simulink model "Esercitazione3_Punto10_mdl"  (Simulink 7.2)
settings: Solver=ode45  StartTime=0.0  StopTime=10.0  RelTol=1e-3
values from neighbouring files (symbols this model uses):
  A = [-6.1   15.4    1.6    [Esercitazione07.m]
  B = [1; 0; 0]    [Esercitazione07.m]
  C = [0 10 10]    [Esercitazione07.m]
  Kyu = -inv(C*inv(A-B*K)*B)    [Esercitazione07.m]
  L = - acker(A',C',[-4 -4 -4])'    [Esercitazione07.m]
  s1 = 5    [Esercitazione07.m]
  s2 = 20    [Esercitazione07.m]
  t1 = 0    [Esercitazione07.m]
  t2 = 10    [Esercitazione07.m]
  X0 = [7 -1 2]'    [Esercitazione07.m]
undefined symbols (not defined in the file or in its folder): K, sd, td

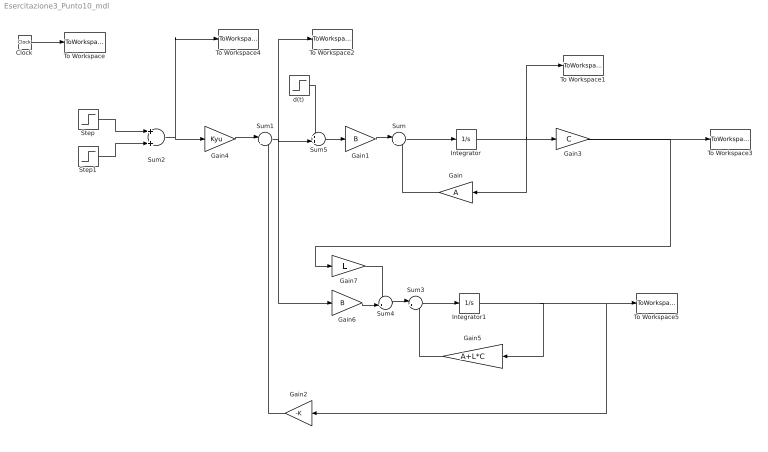
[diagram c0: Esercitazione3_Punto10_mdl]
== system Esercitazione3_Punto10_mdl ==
  Clock : Clock
  Gain : Gain  Orientation=left  Gain=A  Multiplication=Matrix(K*u)  ParameterDataType=sfix(16)  ParameterScaling=2^0  OutDataType=sfix(16)  OutScaling=2^0
  Gain1 : Gain  Gain=B  Multiplication=Matrix(K*u)  ParameterDataType=sfix(16)  ParameterScaling=2^0  OutDataType=sfix(16)  OutScaling=2^0
  Gain2 : Gain  Orientation=left  Gain=-K  Multiplication=Matrix(K*u)  ParameterDataType=sfix(16)  ParameterScaling=2^0  OutDataType=sfix(16)  OutScaling=2^0
  Gain3 : Gain  Gain=C  Multiplication=Matrix(K*u)  ParameterDataType=sfix(16)  ParameterScaling=2^0  OutDataType=sfix(16)  OutScaling=2^0
  Gain4 : Gain  Gain=Kyu  Multiplication=Matrix(K*u)  ParameterDataType=sfix(16)  ParameterScaling=2^0  OutDataType=sfix(16)  OutScaling=2^0
  Gain5 : Gain  Orientation=left  Gain=A+L*C  Multiplication=Matrix(K*u)  ParameterDataType=sfix(16)  ParameterScaling=2^0  OutDataType=sfix(16)  OutScaling=2^0
  Gain6 : Gain  Gain=B  Multiplication=Matrix(K*u)  ParameterDataType=sfix(16)  ParameterScaling=2^0  OutDataType=sfix(16)  OutScaling=2^0
  Gain7 : Gain  Gain=L  Multiplication=Matrix(K*u)  ParameterDataType=sfix(16)  ParameterScaling=2^0  OutDataType=sfix(16)  OutScaling=2^0
  Integrator : Integrator  InitialCondition=X0
  Integrator1 : Integrator  InitialCondition=[0;0;0]
  Step : Step  Time=t1  After=s1  SampleTime=0
  Step1 : Step  Time=t2  After=s2  SampleTime=0
  Sum : Sum  Inputs=|++  OutDataType=sfix(16)  OutScaling=2^0
  Sum1 : Sum  Inputs=|++  OutDataType=sfix(16)  OutScaling=2^0
  Sum2 : Sum  OutDataType=sfix(16)  OutScaling=2^0
  Sum3 : Sum  Inputs=|++  OutDataType=sfix(16)  OutScaling=2^0
  Sum4 : Sum  Inputs=-+|  OutDataType=sfix(16)  OutScaling=2^0
  Sum5 : Sum  Inputs=++|  OutDataType=sfix(16)  OutScaling=2^0
  To Workspace : ToWorkspace  VariableName=time  SampleTime=-1  SaveFormat=Array
  To Workspace1 : ToWorkspace  VariableName=X  SampleTime=-1  SaveFormat=Array
  To Workspace2 : ToWorkspace  VariableName=u  SampleTime=-1  SaveFormat=Array
  To Workspace3 : ToWorkspace  VariableName=y  SampleTime=-1  SaveFormat=Array
  To Workspace4 : ToWorkspace  VariableName=yd  SampleTime=-1  SaveFormat=Array
  To Workspace5 : ToWorkspace  VariableName=X1  SampleTime=-1  SaveFormat=Array
  d(t) : Step  Time=td  After=sd  SampleTime=0
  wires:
  Integrator/1 -> To Workspace1/1, Gain/1, Gain3/1
  Sum/1 -> Integrator/1
  Clock/1 -> To Workspace/1
  Gain3/1 -> To Workspace3/1, Gain7/1
  Gain1/1 -> Sum/1
  Gain/1 -> Sum/2
  Gain4/1 -> Sum1/1
  Sum1/1 -> To Workspace2/1, Gain6/1, Sum5/2
  Gain2/1 -> Sum1/2
  Sum2/1 -> Gain4/1, To Workspace4/1
  Step/1 -> Sum2/1
  Step1/1 -> Sum2/2
  Gain5/1 -> Sum3/2
  Sum3/1 -> Integrator1/1
  Integrator1/1 -> Gain5/1, Gain2/1, To Workspace5/1
  Gain6/1 -> Sum4/2
  Sum4/1 -> Sum3/1
  Gain7/1 -> Sum4/1
  Sum5/1 -> Gain1/1
  d(t)/1 -> Sum5/1
